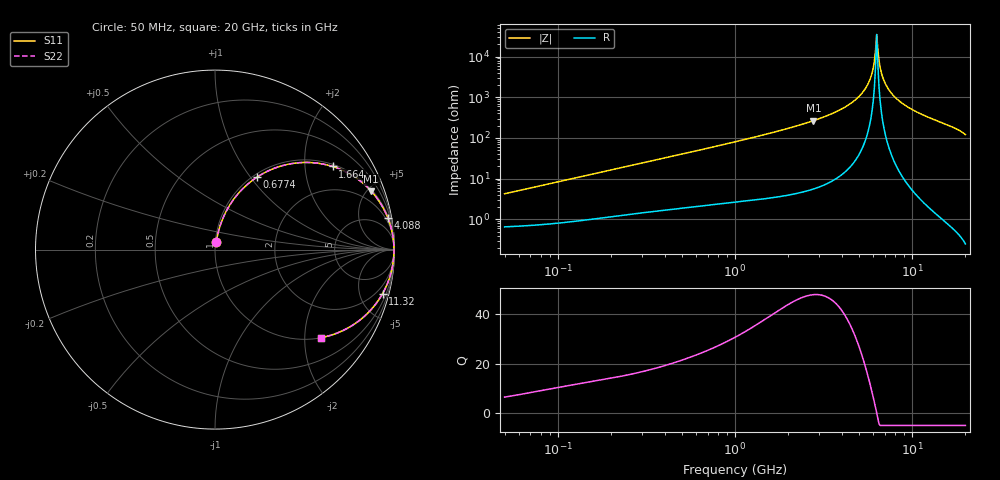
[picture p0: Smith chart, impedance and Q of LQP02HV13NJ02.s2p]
!Murata Part Number: LQP02HV13NJ02
!These Parameters are Measured in Series Mode Connection
!  o--[Z]--o
!Port1  Port2
!  o-------o
!Freq. Start=50[MHz] Stop=20[GHz], 401[Steps]
# Hz S RI R 50
!Freq.(Hz) S11(Real) S11(Imag) S21(Real) S21(Imag) S12(Real) S12(Imag) S22(Real) S22(Imag)
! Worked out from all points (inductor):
!   401 points, 50 MHz to 20 GHz, reference 50 ohm
!   read as one part in series: L = 13.3 nH near 51.52 MHz
!   highest Q = 47.8 at 2.769 GHz (marker M1), where L = 15.2 nH
!   self-resonance near 6.312 GHz
!   S11 on the Smith chart (normalised r, x): 50 MHz: 1.01, +0.08; 677.4 MHz: 1.04, +1.08; 1.664 GHz: 1.07, +2.78; 4.088 GHz: 1, +11; 11.32 GHz: 1.06, -7.62; 20 GHz: 1.00, -2.41
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5e7  0.00821 0.0414  0.9918 -0.0414  0.9918 -0.0414  0.00821 0.0414
1.364002e8  0.0214 0.109  0.9786 -0.109  0.9786 -0.109  0.0214 0.109
3.721004e8  0.094 0.2659  0.906 -0.2659  0.906 -0.2659  0.094 0.2659
6.774326e8  0.2348 0.4042  0.7652 -0.4042  0.7652 -0.4042  0.2348 0.4042
1e9  0.3951 0.4728  0.6049 -0.4728  0.6049 -0.4728  0.3951 0.4728
1.664083e9  0.6551 0.4631  0.3449 -0.4631  0.3449 -0.4631  0.6551 0.4631
2.728004e9  0.8655 0.3309  0.1345 -0.3309  0.1345 -0.3309  0.8655 0.3309
2.769174e9  0.8704 0.3256  0.1296 -0.3256  0.1296 -0.3256  0.8704 0.3256
4.087748e9  0.963 0.1768  0.037 -0.1768  0.037 -0.1768  0.963 0.1768
4.89267e9  0.9853 0.1043  0.0147 -0.1043  0.0147 -0.1043  0.9853 0.1043
5.515528e9  0.9937 0.0555  0.00632 -0.0555  0.00632 -0.0555  0.9937 0.0555
5.856089e9  0.996 0.0311  0.004 -0.0311  0.004 -0.0311  0.996 0.0311
6.034176e9  0.9967 0.0188  0.00331 -0.0188  0.00331 -0.0188  0.9967 0.0188
6.125241e9  0.9969 0.0126  0.00307 -0.0126  0.00307 -0.0126  0.9969 0.0126
6.311513e9  0.9972 0.000344  0.00284 -0.000344  0.00284 -0.000344  0.9972 0.000344
6.503449e9  0.9971 -0.012  0.00291 0.012  0.00291 0.012  0.9971 -0.012
6.802353e9  0.9964 -0.0305  0.0036 0.0305  0.0036 0.0305  0.9964 -0.0305
7.442007e9  0.9929 -0.0677  0.0071 0.0677  0.0071 0.0677  0.9929 -0.0677
8.774992e9  0.9787 -0.1365  0.0213 0.1365  0.0213 0.1365  0.9787 -0.1365
1.131968e10  0.934 -0.2446  0.066 0.2446  0.066 0.2446  0.934 -0.2446
1.621653e10  0.7985 -0.3993  0.2015 0.3993  0.2015 0.3993  0.7985 -0.3993
2e10  0.5911 -0.4906  0.4089 0.4906  0.4089 0.4906  0.5911 -0.4906
